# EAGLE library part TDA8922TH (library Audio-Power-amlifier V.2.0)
The TDA8922C is a high-efficiency Class D audio power amplifier. Typical output power is 2 ´ 75 W with a speaker load impedance of 6 W. The TDA8922C is available in both HSOP24 and DBS23P power packages. The amplifier operates over a wide supply voltage range from ±12.5 V to ±32.5 V and features low quiescent current consumption.
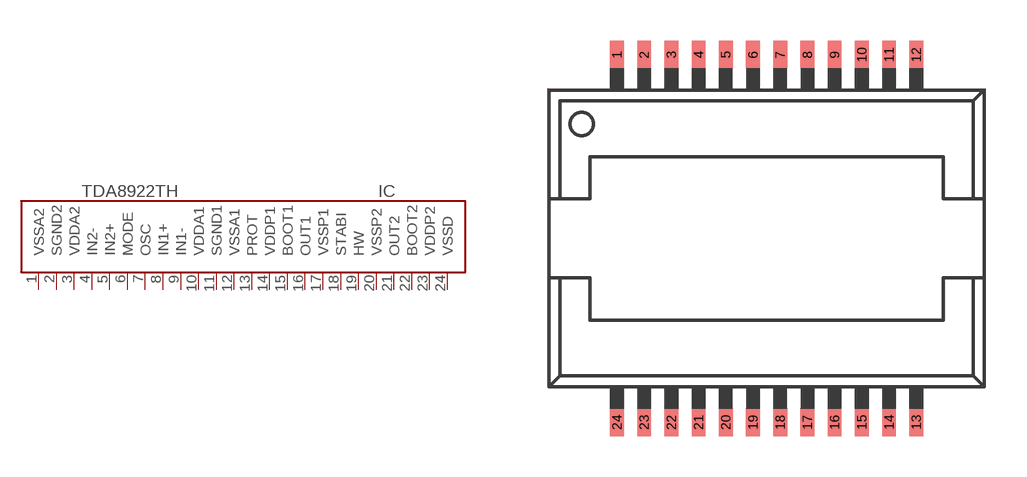
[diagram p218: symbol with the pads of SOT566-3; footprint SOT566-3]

Designator prefix IC

## TDA8922THTDA8922TH  [SOT566-3]
1  VSSA2  pwr
2  SGND2  pwr
3  VDDA2  pwr
4  IN2-  in
5  IN2+  in
6  MODE  in
7  OSC  in
8  IN1+  in
9  IN1-  in
10  VDDA1  pwr
11  SGND1  pwr
12  VSSA1  pwr
13  PROT
14  VDDP1  pwr
15  BOOT1
16  OUT1  out
17  VSSP1  pwr
18  STABI
19  HW
20  VSSP2  pwr
21  OUT2  out
22  BOOT2
23  VDDP2  pwr
24  VSSD  pwr

## Footprint SOT566-3 (pad centres in mm)
smd 0.508 x 1.016: 1 -5.5,6.75; 2 -4.5,6.75; 3 -3.5,6.75; 4 -2.5,6.75; 5 -1.5,6.75; 6 -0.5,6.75; 7 0.5,6.75; 8 1.5,6.75; 9 2.5,6.75; 10 3.5,6.75; 11 4.5,6.75; 12 5.5,6.75; 13 5.5,-6.75; 14 4.5,-6.75; 15 3.5,-6.75; 16 2.5,-6.75; 17 1.5,-6.75; 18 0.5,-6.75; 19 -0.5,-6.75; 20 -1.5,-6.75; 21 -2.5,-6.75; 22 -3.5,-6.75; 23 -4.5,-6.75; 24 -5.5,-6.75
